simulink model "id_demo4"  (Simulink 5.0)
settings: Solver=ode45  SolverMode=SingleTasking  StartTime=0.0  StopTime=10  RelTol=1e-3  AbsTol=1e-3

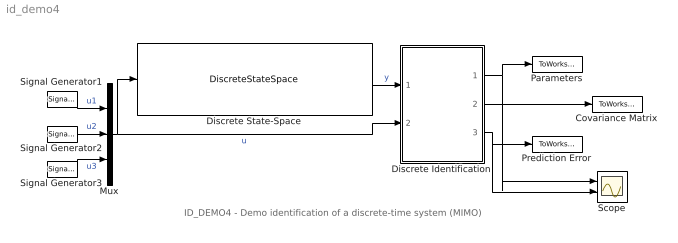
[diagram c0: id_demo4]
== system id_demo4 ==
  note: ID_DEMO4 - Demo identification of a discrete-time system (MIMO)
  Covariance Matrix : ToWorkspace  VariableName=CovMatrix  SaveFormat=Array
  Discrete Identification : Subsystem  mask(Discrete Identification){par3=[3,2], par1=[2,1], Ds=[0], par2=[0.985,0.01], poc=zeros(1,16), kov=[10e6], ts=[1]}
      mask prompts: par3 "Number of inputs and outputs -  [in,out]:"; par1 "Degrees of numerator and denominator -  [dn, dd]:"; Ds "Discrete time delay - [D]:"; par2 "Exponential forgetting and Bittanti's correction - [L, d]:"; poc "Initial parameter estimates - [theta(1) ... theta(n)]:"; kov "Covariance matrix (see help, standard - [10e6]):"; ts "Sampling time - [ts]:"
      mask help: Discrete identification Authors: Lubos Cirka and Miroslav Fikar 1998 - 2006
      mask init:
      | % State-space realisation of discete-time filters
      | %
      | % Input:
      | %    y_1(k), ..., y_in(k), u_1(k), ..., u_out(k)
      | % Output:
      | %    y_1(k), ..., y_in(k), -y_1(k-1), ..., -y_in(k-1), -y_1(k-2), ..., -y_in(k-2), ..., 
      | %    u_1(k), ..., u_out(k), u_1(k-1), ..., u_out'(k-1), u_1(k-2), ..., u_out(k-2), ...
      | 
      | % Parameters definition
      | cit = par1(1); % numerator degree 
      | men = par1(2); % denumerator degree
      | L = par2(1); % exponential forgetting
      | d = par2(2); % Bittanti's correction
      | n = cit*par3(1)+men*par3(2); % number of data
      | m = par3(2); % 
      | in = par3(1); % number of inputs
      | out = par3(2); % number of outputs
      | 
      | % State-space realisation of the output filter
      | A0=zeros(men*out);
      | A0(out+1:men*out,1:(men-1)*out)=eye((men-1)*out);
      | Ay=A0;
      | 
      | B0=-eye(out);
      | B1=zeros((men-1)*out,out);
      | By=[B0;B1];
      | 
      | C0=zeros(out,men*out);
      | C1=eye(men*out);
      | Cy=[C0;C1];
      | 
      | D1=eye(out);
      | D2=zeros(men*out,out);
      | Dy=[D1;D2];
      | 
      | % State-space realisation of the input filter
      | 
      | a0=zeros(in,(cit+Ds)*in);
      | a1=eye((cit+Ds-1)*in);
      | a2=zeros((cit+Ds-1)*in,in);
      | Au=[a0;[a1 a2]];
      | 
      | b0=eye(in);
      | b1=zeros((cit+Ds-1)*in,in);
      | Bu=[b0;b1];
      | 
      | c0=zeros(cit*in,Ds*in);
      | c1=eye(cit*in);
      | Cu=[c0 c1];
      | 
      | Du=zeros(cit*in,in);
  Discrete State-Space : DiscreteStateSpace  A=[-0.1 1 -0.2 0;0 0 0 0;-0.3 0 -0.4 1;0 0 0 0]  B=[1.1 1.3 1.5;1.2 1.4 1.6;2.1 2.3 2.5;2.2 2.4 2.6]  C=[1 0 0 0;0 0 1 0]  D=[0 0 0;0 0 0]
  Mux : Mux  Inputs=3
  Parameters : ToWorkspace  VariableName=AB  SaveFormat=Array
  Prediction Error : ToWorkspace  VariableName=PredError  SaveFormat=Array
  Scope : Scope  NumInputPorts=2
  Signal Generator1 : SignalGenerator  Units=rad/sec
  Signal Generator2 : SignalGenerator  WaveForm=square  Frequency=2  Units=rad/sec
  Signal Generator3 : SignalGenerator  WaveForm=square  Frequency=2  Units=rad/sec
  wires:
  Discrete State-Space/1 -> Discrete Identification/1(y)  "y"
  Mux/1 -> Discrete Identification/2(u), Discrete State-Space/1  "u"
  Discrete Identification/1(B) -> Scope/1, Parameters/1
  Discrete Identification/2("Covariance matrix ") -> Covariance Matrix/1
  Discrete Identification/3(prediction error) -> Prediction Error/1, Scope/2
  Signal Generator1/1 -> Mux/1  "u1"
  Signal Generator2/1 -> Mux/2  "u2"
  Signal Generator3/1 -> Mux/3  "u3"

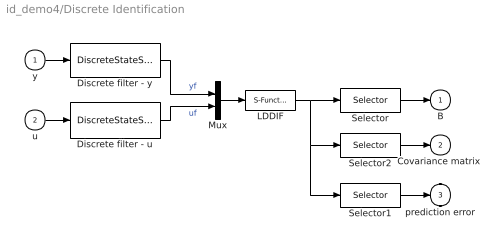
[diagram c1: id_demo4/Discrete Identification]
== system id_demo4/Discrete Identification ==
  y : Inport
  u : Inport  Port=2
  Discrete filter - u : DiscreteStateSpace  A=Au  B=Bu  C=Cu  D=Du  SampleTime=ts
  Discrete filter - y : DiscreteStateSpace  A=Ay  B=By  C=Cy  D=Dy  SampleTime=ts
  LDDIF : S-Function  FunctionName=lddif_s  Parameters=m, n, L, d, poc, kov, ts
  Mux : Mux  Inputs=2
  Selector : Selector  Elements=[1:1:n*m]  InputPortWidth=n*m+n*n+m
  Selector1 : Selector  Elements=[n*m+n*n+1:1:n*m+n*n+m]  InputPortWidth=n*m+n*n+m
  Selector2 : Selector  Elements=[n*m+1:1:n*m+n*n]  InputPortWidth=n*m+n*n+m
  B : Outport  InitialOutput=0
  "Covariance matrix " : Outport  Port=2  InitialOutput=0
  prediction error : Outport  Port=3  InitialOutput=0
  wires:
  Selector1/1 -> prediction error/1
  Selector2/1 -> "Covariance matrix "/1
  Mux/1 -> LDDIF/1
  Selector/1 -> B/1
  y/1 -> Discrete filter - y/1
  u/1 -> Discrete filter - u/1
  Discrete filter - y/1 -> Mux/1  "yf"
  Discrete filter - u/1 -> Mux/2  "uf"
  LDDIF/1 -> Selector2/1, Selector1/1, Selector/1
